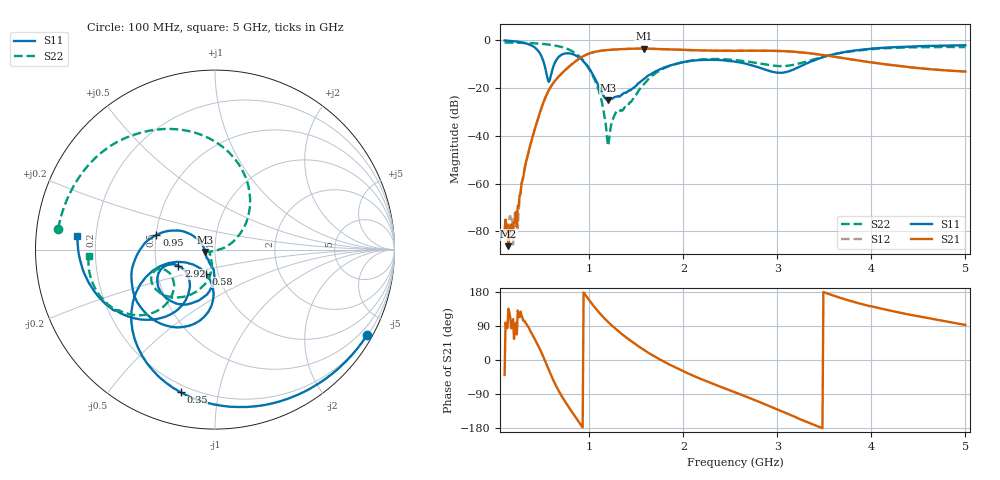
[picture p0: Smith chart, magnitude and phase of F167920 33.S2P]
!  2-Port S-parameters saved by WinCal
! VAR MeasName=S-Parameters (CALIBRATED_DATA) read from VNA (N5242A)
! VAR MeasDate=2016-11-22 9:56:51
! VAR NAME=F167920 33
! VAR FILENAME=F167920 33.S2P
! VAR DATE=2016-11-22 9:56:51
! VAR PHYS_PORTS=1,2
# Hz S DB R 50
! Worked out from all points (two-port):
!   491 points, 100 MHz to 5 GHz, reference 50 ohm
!   highest |S21| = -3.65 dB at 1.58 GHz (marker M1); lowest = -86.1 dB at 140 MHz (marker M2)
!   |S21| within 3 dB of the highest: 945.3 MHz to 3.542 GHz (2.597 GHz wide, 116 % of centre)
!   lowest |S11| = -25.2 dB at 1.2 GHz (marker M3), VSWR 1.12, Z = 44.9 - j1.16 ohm
!   |S11| at or under -10 dB: 520.5 MHz to 629.6 MHz (109.1 MHz wide, 19 % of centre); 962.3 MHz to 1.927 GHz (964.7 MHz wide, 66.8 % of centre); 2.668 GHz to 3.302 GHz (634.1 MHz wide, 21.2 % of centre)
!   |S22| runs from -44.3 to -1.1 dB; largest |S21 - S12| = 0.0017
!   S11 on the Smith chart (normalised r, x): 100 MHz: 0.22, -3.82; 350 MHz: 0.16, -0.77; 580 MHz: 0.87, -0.24; 950 MHz: 0.50, +0.09; 2.92 GHz: 0.65, -0.12; 5 GHz: 0.13, +0.05
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1e8  -0.25 -29.3  -79.50 -39.5  -79.76 150.1  -1.10 172.4
1.4e8  -0.36 -40.7  -86.15 135.3  -80.20 84.9  -1.12 169.3
2.1e8  -0.63 -60.9  -76.16 80.7  -71.57 87.6  -1.18 163.9
2.4e8  -0.78 -69.7  -69.34 130.7  -78.79 115.0  -1.20 161.5
3.5e8  -1.75 -103.6  -47.44 88.1  -47.69 86.9  -1.33 152.2
4.6e8  -4.75 -143.5  -32.17 36.4  -32.17 36.7  -1.54 141.4
5.8e8  -16.81 -110.1  -20.30 -31.9  -20.29 -31.9  -2.03 127.2
7.1e8  -6.13 -119.3  -13.90 -96.4  -13.89 -96.4  -3.03 108.0
8.1e8  -5.80 -152.7  -10.33 -134.7  -10.31 -134.7  -4.55 88.6
9.2e8  -8.17 174.2  -7.17 -174.2  -7.16 -174.2  -7.93 62.4
9.5e8  -9.45 166.1  -6.55 175.0  -6.55 174.9  -9.30 55.2
1.1e9  -19.26 149.7  -4.69 126.6  -4.69 126.6  -21.09 19.8
1.2e9  -25.24 -166.4  -4.21 100.3  -4.22 100.3  -44.29 -72.6
1.29e9  -23.71 -135.5  -3.98 80.3  -3.97 80.3  -30.02 -156.8
1.58e9  -16.39 -91.2  -3.65 27.0  -3.65 27.0  -18.59 -100.3
1.74e9  -12.49 -98.0  -3.82 2.9  -3.82 2.9  -13.05 -109.4
2.12e9  -8.59 -127.0  -4.33 -43.1  -4.32 -43.1  -8.46 -137.2
2.55e9  -9.09 -155.3  -4.55 -85.3  -4.55 -85.3  -8.42 -158.1
2.92e9  -13.03 -156.1  -4.55 -121.9  -4.55 -121.9  -10.57 -156.9
3.37e9  -8.87 -120.6  -5.72 -169.2  -5.71 -169.2  -8.34 -132.0
4.19e9  -3.15 -157.0  -10.43 130.9  -10.41 130.7  -3.43 -153.8
5e9  -2.27 174.4  -13.23 92.5  -13.23 92.3  -3.04 -176.9
